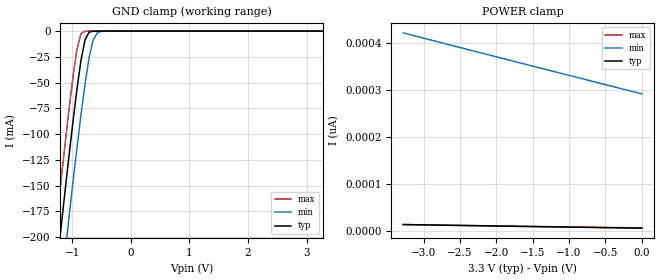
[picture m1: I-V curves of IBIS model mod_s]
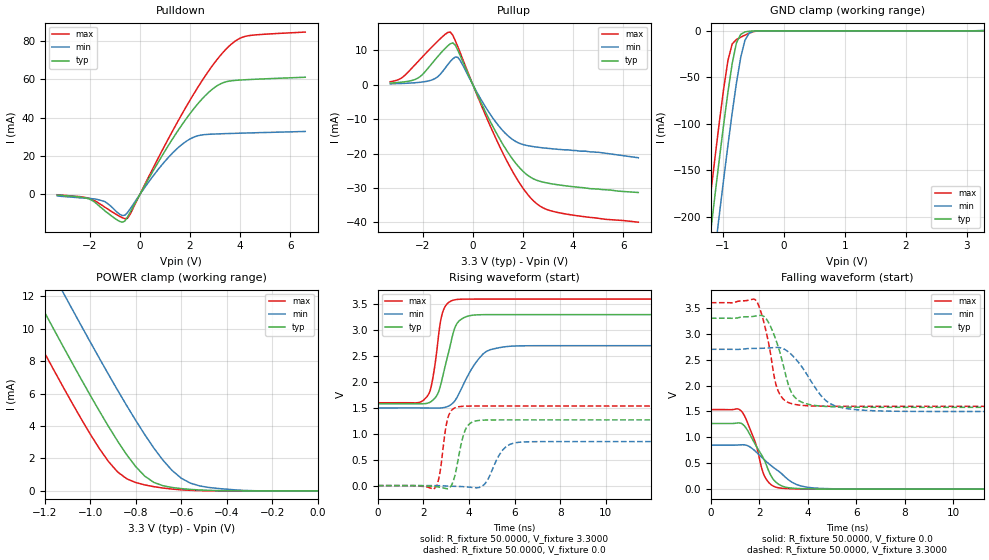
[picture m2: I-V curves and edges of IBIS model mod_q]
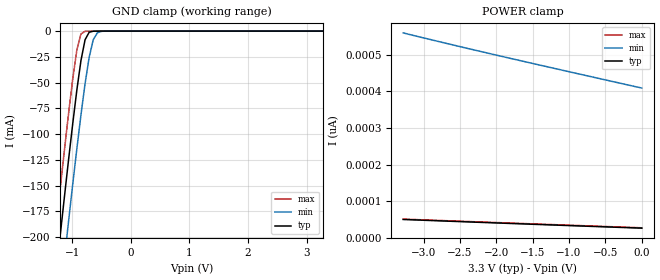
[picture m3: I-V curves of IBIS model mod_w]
| IBIS (I/O, Buffer, Information, Specification) Model, officially
| electronic behavioral standard for Buffer structures of digital pins.
[IBIS ver]  4.0
[File name] m95xxx_g11_tssop8.ibs
[File Rev]  1.0
[Date]   10 Oct 2015
[Source]   CAD & Design Services (Catania) - STMicroelectronics
[Notes]
   (Note1)  This IBIS model includes the TSSOP8 ceramic package parasitic data
   (Note2)  This IBIS model considers: VCC=3.30(TYP), 2.70(MIN), 3.60(MAX)
   (Note3)  This IBIS model has some Notes about the non-monotonicity
   of the I-V curves, but they are not indicative of problems
   inside the model;
[Copyright] (c) 2015 STMicroelectronics
|   Component M95XXX
[Component] M95XXX
[Manufacturer] STMicroelectronics
[Package]
| variable  typ   min   max
R_pkg   0.0   0.0   0.0
L_pkg   0.0H   0.0H   0.0H
C_pkg   0.0F   0.0F   0.0F
[Pin]   signal_name   model_name   R_pin   L_pin   C_pin
1   SN   mod_s   NA   NA   NA
2   Q   mod_q   NA   NA   NA
3   WN   mod_w   NA   NA   NA
4   GND   GND   NA   NA   NA
5   D   mod_s   NA   NA   NA
6   C   mod_s   NA   NA   NA
7   HOLDN   mod_h   NA   NA   NA
8   VCC   POWER   NA   NA   NA
[Package Model]  182696_TSSOP8
[Define Package Model]  182696_TSSOP8
[Manufacturer]  STMicroelectronics
[OEM]  STMicroelectronics
[Description]  8 pin TSSOP package
[Number Of Pins]  8
[Pin Numbers]
|Pin Num   Terminal Name
1   | net1
2   | net2
3   | net3
4   | net4_GND
5   | net5
6   | net6
7   | net7
8   | net8_VDD
[Model Data]
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[End Model Data]
[End Package Model]
| Models and submodels in the file (4): mod_s (Input), mod_q (I/O), mod_w (Input), mod_h (Input)
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|   Model mod_s
[Model]   mod_s
Model_type Input
Vinl   =   1.000V
Vinh   =   2.300V
C_comp   2.119pF   2.024pF   2.323pF
[Temperature Range]  25.0000   0.1050k   -40.0000
[Voltage Range]   3.3000V   2.7000V   3.6000V
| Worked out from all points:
|   GND clamp passes 1 mA (typ) near -0.70 V on its own axis
[GND_clamp]
|Voltage   I(typ)   I(min)   I(max)
-3.3V     -1.355A    -1.412A    -1.313A
-1.34V    -270.3mA   -330.7mA   -224.8mA
-1.27V    -233mA     -293.4mA   -187.4mA
-1.2V     -196.1mA   -256.5mA   -150.5mA
-1.13V    -159.7mA   -219.9mA   -114.2mA
-1.06V    -124.1mA   -183.9mA   -79.16mA
-920mV    -57.12mA   -114.2mA   -18.15mA
-850mV    -28.51mA   -81.35mA   -2.609mA
-780mV    -8.357mA   -51.08mA   -131.1uA
-640mV    -95.71uA   -8.329mA   -224.5nA
-500mV    -655.8nA   -243.4uA   -381.5pA
3.28V     6.871pA    315.5pA    6.69pA
[POWER_clamp]
|Voltage   I(typ)   I(min)   I(max)
-3.28V    14.67pA    422.5pA    14.54pA
-2.52V    12.77pA    392.2pA    12.82pA
-1.44V    10.18pA    349.4pA    10.44pA
0V        6.915pA    292.7pA    7.361pA
|   Model mod_q
[Model]   mod_q
Model_type I/O
Enable   Active-Low
Vinl   =   1.000V
Vinh   =   2.300V
Vmeas  =   1.650V
Cref   =   30pF
C_comp   2.925pF   2.668pF   3.207pF
[Temperature Range]  25.0000   0.1050k   -40.0000
[Voltage Range]   3.3000V   2.7000V   3.6000V
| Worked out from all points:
|   slope of the pulldown table from 0 to 0.495 V, typ, clamps not added: 43.1 ohm
|   slope of the pullup table from 0 to 0.495 V, typ, clamps not added: 63.8 ohm
|   GND clamp passes 1 mA (typ) near -0.63 V on its own axis
|   POWER clamp passes 1 mA (typ) near -0.77 V on its own axis
|   rising waveform, R_fixture 50.0000, V_fixture 3.3000: 20-80 % time 569ps typ, 932ps min, 383ps max; typ from 1.58 V to 3.3 V
|   rising waveform, R_fixture 50.0000, V_fixture 0.0: 20-80 % time 373ps typ, 576ps min, 284ps max; typ from 0 V to 1.27 V
|   falling waveform, R_fixture 50.0000, V_fixture 0.0: 20-80 % time 830ps typ, 1.28ns min, 604ps max; typ from 1.27 V to 0 V
|   falling waveform, R_fixture 50.0000, V_fixture 3.3000: 20-80 % time 642ps typ, 1.09ns min, 501ps max; typ from 3.3 V to 1.58 V
[Pulldown]
|Voltage   I(typ)   I(min)   I(max)
-3.3V     -300uA     -760uA     -144uA
-2V       -2.5mA     -2.1mA     -2mA
-1.4V     -8.5mA     -3.7mA     -6.6mA
-800mV    -14.04mA   -10.33mA   -11.44mA
-600mV    -13.83mA   -10.79mA   -12.57mA
-500mV    -11.87mA   -9.519mA   -12.47mA
800mV     18.29mA    14.16mA    20.66mA
1.7V      36.68mA    26.26mA    42.35mA
2.6V      51.34mA    31.18mA    61.55mA
3.4V      58.52mA    31.67mA    75.13mA
4.2V      59.72mA    31.99mA    82.29mA
6.6V      61.03mA    32.81mA    84.54mA
[Pullup]
|Voltage   I(typ)   I(min)   I(max)
-3.3V     521uA      294uA      909uA
-2.8V     806uA      405uA      2.235mA
-2.2V     1.926mA    670uA      6.685mA
-1.5V     7.375mA    1.868mA    12mA
-900mV    11.94mA    6.803mA    15.33mA
-600mV    10.01mA    7.993mA    11.03mA
500mV     -7.834mA   -6.397mA   -8.779mA
1.3V      -18.54mA   -14.14mA   -21.36mA
1.9V      -24.41mA   -17.13mA   -29mA
2.4V      -27.28mA   -17.95mA   -33.61mA
3.4V      -29.07mA   -18.75mA   -37.13mA
6.6V      -31.3mA    -21.2mA    -39.93mA
[GND_clamp]
|Voltage   I(typ)   I(min)   I(max)
-3.3V     -1.448A    -1.504A    -1.412A
-1.27V    -253.9mA   -314.2mA   -213.5mA
-1.2V     -214.5mA   -274.9mA   -174.1mA
-1.13V    -175.7mA   -236mA     -135.4mA
-1.06V    -137.7mA   -197.6mA   -97.89mA
-920mV    -66.08mA   -123.4mA   -32.04mA
-850mV    -35.23mA   -88.39mA   -14.1mA
-780mV    -12.93mA   -56.07mA   -9.262mA
-710mV    -3.708mA   -28.61mA   -6.819mA
-640mV    -1.177mA   -9.975mA   -4.574mA
-430mV    -26.05uA   -158.4uA   -67.99uA
3.28V     145.8pA    614.2uA    123.1pA
[POWER_clamp]
|Voltage   I(typ)   I(min)   I(max)
-3.28V    67.55mA    70.7mA     65.16mA
-1.36V    15.21mA    18.54mA    12.69mA
-1.32V    14.15mA    17.49mA    11.63mA
-1.24V    12.04mA    15.38mA    9.521mA
-1.12V    8.922mA    12.25mA    6.427mA
-960mV    4.924mA    8.178mA    2.612mA
-880mV    3.078mA    6.217mA    1.172mA
-760mV    906.8uA    3.463mA    369.2uA
-680mV    319uA      1.891mA    177.9uA
-600mV    143uA      786uA      68.21uA
-440mV    18.61uA    152.6uA    2.435uA
0V        149.9pA    1.374nA    157.9pA
[Ramp]
| variable   typ   min   max
dV/dt_r  0.7610/0.4103n   0.5095/0.6320n   0.9211/0.3567n
dV/dt_f  1.0304/0.7213n   0.7210/1.2280n   1.2006/0.5636n
R_load = 50.0000
[Rising Waveform]
R_fixture= 50.0000
V_fixture= 3.3000
V_fixture_min= 2.7000
V_fixture_max= 3.6000
|time   V(typ)   V(min)   V(max)
0s        1.58V      1.499V     1.599V
2.16ns    1.588V     1.498V     1.717V
2.4ns     1.643V     1.497V     2.044V
2.64ns    1.784V     1.496V     2.806V
2.82ns    2.056V     1.501V     3.307V
3.3ns     2.935V     1.596V     3.577V
3.66ns    3.211V     1.865V     3.597V
4.47ns    3.297V     2.471V     3.6V
5.22ns    3.3V       2.652V     3.6V
15ns      3.3V       2.7V       3.6V
[Rising Waveform]
R_fixture= 50.0000
V_fixture= 0.0
V_fixture_min= 0.0
V_fixture_max= 0.0
|time   V(typ)   V(min)   V(max)
0s        5.101nV    210.2nV    5.035nV
2.46ns    -16.65mV   97.6uV     -68.49mV
2.685ns   -27.65mV   -1.595mV   159.4mV
3.075ns   -59.31mV   -8.882mV   1.31V
3.495ns   438.1mV    -15.01mV   1.517V
3.855ns   1.092V     -23.88mV   1.534V
4.335ns   1.251V     -42.61mV   1.536V
5.445ns   1.268V     671.5mV    1.536V
5.985ns   1.268V     822.6mV    1.536V
15ns      1.268V     849.2mV    1.536V
[Falling Waveform]
R_fixture= 50.0000
V_fixture= 0.0
V_fixture_min= 0.0
V_fixture_max= 0.0
|time   V(typ)   V(min)   V(max)
0s        1.268V     849.2mV    1.536V
1.08ns    1.276V     851.1mV    1.553V
1.275ns   1.264V     857mV      1.496V
1.815ns   877.7mV    740.2mV    926.3mV
2.205ns   559.4mV    567.2mV    259.5mV
2.475ns   262.8mV    457.7mV    90.33mV
2.745ns   110.9mV    362.6mV    30.78mV
3.39ns    18.21mV    121.6mV    6.25mV
4.245ns   4.013mV    22.62mV    786.7uV
15ns      -6.325nV   236.2nV    2.777nV
[Falling Waveform]
R_fixture= 50.0000
V_fixture= 3.3000
V_fixture_min= 2.7000
V_fixture_max= 3.6000
|time   V(typ)   V(min)   V(max)
0s        3.3V       2.7V       3.6V
1.875ns   3.344V     2.718V     3.634V
2.235ns   3.314V     2.722V     3.127V
2.73ns    2.817V     2.736V     1.95V
2.985ns   2.394V     2.711V     1.74V
3.315ns   1.874V     2.602V     1.653V
3.735ns   1.681V     2.373V     1.619V
4.725ns   1.597V     1.715V     1.601V
5.445ns   1.585V     1.569V     1.599V
15ns      1.58V      1.499V     1.599V
|   Model mod_w
[Model]   mod_w
Model_type Input
Vinl   =   1.000V
Vinh   =   2.300V
C_comp   2.119pF   2.024pF   2.323pF
[Temperature Range]  25.0000   0.1050k   -40.0000
[Voltage Range]   3.3000V   2.7000V   3.6000V
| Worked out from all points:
|   GND clamp passes 1 mA (typ) near -0.70 V on its own axis
[GND_clamp]
|Voltage   I(typ)   I(min)   I(max)
-3.3V     -1.356A    -1.413A    -1.314A
-1.34V    -270.6mA   -330.9mA   -225.1mA
-1.27V    -233.3mA   -293.6mA   -187.7mA
-1.2V     -196.3mA   -256.7mA   -150.7mA
-1.13V    -159.9mA   -220.1mA   -114.5mA
-1.06V    -124.2mA   -184mA     -79.35mA
-920mV    -57.23mA   -114.3mA   -18.3mA
-850mV    -28.6mA    -81.43mA   -2.741mA
-780mV    -8.431mA   -51.14mA   -241.4uA
-640mV    -131.4uA   -8.363mA   -67.87uA
-500mV    -8.308uA   -254.9uA   -28.04uA
3.28V     25.49pA    435.3pA    24.34pA
[POWER_clamp]
|Voltage   I(typ)   I(min)   I(max)
-3.28V    49.42pA    560.5pA    50.46pA
-2.88V    46.41pA    541pA      47.49pA
-2V       39.92pA    499.6pA    41.03pA
0V        25.63pA    409.4pA    26.62pA
